[IBIS Ver]   3.2
[File Name]   sprm125.ibs
[File Rev]   0.1
[Date]   September 5, 2003
[Source]   IBIS Model Generated from PACED 4.51F
[Disclaimer]   Please be aware that in the absence of a written agreement
|   Texas Instruments(TI) assumes no liability for:
|   (1) The accuracy of the IBIS models provided to your company
|   (2) The proper functioning of these Models in your design
|   or for any resulting applications
|   (3) Infringement of patents, copyrights or intellectual
|   property rights resulting from your use of these
|   models.
|   TI provides IBIS Models as a service to our customers and
|   therefore reserves the right to limit distribution of the
|   Models.
[Copyright]   Property of Texas Instruments Incorporated.
|   Unauthorized reproduction and/or distribution is strictly.
|   prohibited.
|   This product is protected under copyright law and trade
|   secret law as an unpublished work.
|   Created 2003,(C) Copyright 1999-2003,
|   Texas Instruments Incorporated., All Rights Reserved.
|   These commodities are under the U.S. Government
|   distribution license control. As such,they are not to be
|   re-exported without the prior approval of the U.S.
|   Department of Commerce.
[Notes]
|****** ****   ***** *****   ******  Package Models  **************************
[Component]   DM641_GDK
[Manufacturer]  Texas Instruments
[Package]
|Variable  Typ   Min   Max
 R_pkg   0.12581866  0.0708   0.1927
 L_pkg   2.32E-09   1.26E-09  3.57E-09
 C_pkg   1.14E-12   6.40E-13  1.77E-12
[Pin]   signal_name  model_name   R_pin   L_pin   C_pin
B4   NMI   IT33THYPD   0.1574   2.92E-09  1.37E-12
A4   TINP0   IT33THYPD   0.1714   3.17E-09  1.50E-12
C5   TOUT0   BT3325CTPD   0.1355   2.49E-09  1.22E-12
B5   TOUT1   BT3325CTPU   0.1504   2.77E-09  1.35E-12
A5   TINP1   IT33THYPD   0.1652   3.05E-09  1.47E-12
D6   CLKOUT4   BT3315DTHYPU   0.1173   2.16E-09  1.06E-12
C6   CLKOUT6   BT3315DTHYPU   0.1352   2.50E-09  1.19E-12
A15   EMU0   BT3315DTHYPU   0.1531   2.82E-09  1.33E-12
A16   TCK   IT33THYPU   0.1598   2.93E-09  1.43E-12
C14   EMU1   BT3315DTHYPU   0.1107   2.01E-09  1.02E-12
B15   EMU2   BT3315DTHYPU   0.1318   2.37E-09  1.17E-12
C15   EMU3   BT3315DTHYPU   0.1149   2.09E-09  1.06E-12
D14   TRSTZ   IT33THYPD   0.0895   1.61E-09  8.52E-13
B16   EMU5   BT3315DTHYPU   0.1348   2.46E-09  1.21E-12
A17   EMU7   BT3315DTHYPU   0.1482   2.72E-09  1.32E-12
C16   EMU6   BT3315DTHYPU   0.1043   1.89E-09  9.63E-13
D15   EMU4   BT3315DTHYPU   0.0836   1.51E-09  7.86E-13
E15   TMS   IT33THYPU   0.0754   1.35E-09  7.23E-13
B17   EMU9   BT3315DTHYPU   0.1316   2.41E-09  1.18E-12
A18   TDI   IT33THYPU   0.1516   2.78E-09  1.35E-12
C17   EMU10   BT3315DTHYPU   0.1174   2.15E-09  1.05E-12
D16   EMU8   BT3315DTHYPU   0.093   1.70E-09  8.42E-13
B18   TDO   BT3325CTPU   0.1357   2.49E-09  1.22E-12
A20   AED13   BT3315DTPU   0.1718   3.17E-09  1.51E-12
B20   AED11   BT3315DTPU   0.1583   2.93E-09  1.39E-12
D17   EMU11   BT3315DTHYPU   0.0955   1.75E-09  8.81E-13
C19   AED15   BT3315DTPU   0.1283   2.36E-09  1.16E-12
A21   AED09   BT3315DTPU   0.174   3.21E-09  1.54E-12
C20   AED10   BT3315DTPU   0.1378   2.53E-09  1.26E-12
B21   AED07   BT3315DTPU   0.1588   2.93E-09  1.42E-12
D19   AED14   BT3315DTPU   0.1105   2.01E-09  1.04E-12
C21   AED06   BT3315DTPU   0.1445   2.64E-09  1.33E-12
B22   AED03   BT3315DTPU   0.1665   3.06E-09  1.51E-12
D20   AED12   BT3315DTPU   0.1178   2.14E-09  1.11E-12
A23   AED05   BT3315DTPU   0.1861   3.43E-09  1.67E-12
C22   AED04   BT3315DTPU   0.1485   2.71E-09  1.37E-12
D21   AED08   BT3315DTPU   0.1256   2.29E-09  1.17E-12
B23   AED02   BT3315DTPU   0.1627   3.00E-09  1.44E-12
A24   AED01   BT3315DTPU   0.1927   3.57E-09  1.68E-12
B24   AED00   BT3315DTPU   0.1784   3.29E-09  1.59E-12
C25   AED30   BT3315DTPU   0.1772   3.27E-09  1.57E-12
C26   AED31   BT3315DTPU   0.1873   3.44E-09  1.66E-12
D25   AED28   BT3315DTPU   0.161   2.97E-09  1.47E-12
D26   AED29   BT3315DTPU   0.1818   3.39E-09  1.71E-12
E25   AED26   BT3315DTPU   0.1682   3.14E-09  1.57E-12
E24   AED27   BT3315DTPU   0.1418   2.60E-09  1.29E-12
F26   AED22   BT3315DTPU   0.1743   3.21E-09  1.55E-12
F25   AED24   BT3315DTPU   0.1589   2.91E-09  1.42E-12
F24   AED25   BT3315DTPU   0.1434   2.63E-09  1.29E-12
F23   AED23   BT3315DTPU   0.1237   2.25E-09  1.12E-12
G26   AED18   BT3315DTPU   0.1471   2.70E-09  1.31E-12
G25   AED20   BT3315DTPU   0.1445   2.64E-09  1.30E-12
G24   AED21   BT3315DTPU   0.1401   2.57E-09  1.26E-12
G23   AED19   BT3315DTPU   0.1202   2.20E-09  1.08E-12
H25   AECLKIN   IT33THYPD   0.1487   2.75E-09  1.29E-12
H24   AED16   BT3315DTPU   0.1248   2.30E-09  1.09E-12
H23   AED17   BT3315DTPU   0.1074   1.97E-09  9.56E-13
J25   ASDCASZ   BT3315DTPU   0.1364   2.48E-09  1.17E-12
J24   ASDRASZ   BT3315DTPU   0.1224   2.24E-09  1.03E-12
J23   AECLKOT2   BT3315DTPD   0.1   1.86E-09  8.55E-13
J26   AECLKOT1   BT3315DTPD   0.1448   2.65E-09  1.23E-12
K23   ACE2Z   BT3315DTPU   0.0938   1.72E-09  8.52E-13
K24   ACE1Z   BT3315DTPU   0.1113   2.04E-09  1.02E-12
K25   ACE0Z   BT3315DTPU   0.1259   2.31E-09  1.15E-12
K26   ASDWEZ   BT3315DTPU   0.1406   2.59E-09  1.26E-12
L23   ABE01Z   BT3315DTPU   0.0961   1.75E-09  8.81E-13
L22   AARDY   IT33THYPU   0.0784   1.42E-09  7.32E-13
L24   ABE00Z   BT3315DTPU   0.1071   1.97E-09  9.65E-13
L25   ASDCKE   BT3315DTPU   0.125   2.30E-09  1.12E-12
L26   ACE3Z   BT3315DTPU   0.139   2.56E-09  1.23E-12
M22   APDTZ   BT3315DTPU   0.074   1.34E-09  6.98E-13
M23   AEA04   BT3315DTPD   0.0903   1.64E-09  8.30E-13
M24   AEA03   BT3315DTPD   0.105   1.91E-09  9.64E-13
M25   ABE03Z   BT3315DTPU   0.1201   2.20E-09  1.08E-12
N22   AHOLDAZ   BT3315DTPU   0.0724   1.30E-09  6.85E-13
N23   AEA07   BT3315DTPD   0.1669   3.04E-09  1.52E-12
N24   AEA06   BT3315DTPD   0.1016   1.84E-09  9.39E-13
M26   ABE02Z   BT3315DTPU   0.1409   2.59E-09  1.26E-12
N26   AEA05   BT3315DTPD   0.1326   2.42E-09  1.20E-12
P26   AEA08   BT3315DTPD   0.1329   2.42E-09  1.20E-12
P24   AEA09   BT3315DTPD   0.103   1.87E-09  9.43E-13
P23   AEA10   BT3315DTPD   0.0883   1.60E-09  8.14E-13
P22   ABUSREQ0   BT3315DTPU   0.0734   1.33E-09  6.83E-13
R24   AEA11   BT3315DTPD   0.1062   1.94E-09  9.60E-13
R23   AEA12   BT3315DTPD   0.0913   1.67E-09  8.28E-13
R22   ASOE3Z   BT3315DTPU   0.0749   1.36E-09  6.97E-13
T25   AEA13   BT3315DTPD   0.1263   2.32E-09  1.11E-12
T24   AEA14   BT3315DTPD   0.1116   2.05E-09  9.87E-13
U26   AEA15   BT3315DTPD   0.1406   2.61E-09  1.22E-12
U25   AEA16   BT3315DTPD   0.1258   2.32E-09  1.13E-12
U24   AEA17   BT3315DTPD   0.1112   2.05E-09  9.99E-13
U23   AEA22   BT3315DTPD   0.0967   1.77E-09  8.72E-13
V26   AEA19   BT3315DTPD   0.14   2.63E-09  1.28E-12
V25   AEA20   BT3315DTPD   0.1264   2.36E-09  1.16E-12
V24   AEA21   BT3315DTPD   0.1128   2.10E-09  1.03E-12
V23   AEA18   BT3315DTPD   0.0992   1.83E-09  8.94E-13
W24   AHOLDZ   IT33THYPU   0.121   2.23E-09  1.07E-12
AC17   VP0CTL1   BT3325CTHYPD   0.099   1.83E-09  9.31E-13
AD17   VP0CTL2   BT3325CTHYPD   0.1128   2.08E-09  1.03E-12
AE17   VP0CTL0   BT3325CTHYPD   0.1271   2.35E-09  1.16E-12
AF17   VP0D00   BT3325CTHYPD   0.1412   2.61E-09  1.23E-12
AB16   VP0D05   BT3325CTHYPD   0.0792   1.45E-09  7.33E-13
AC16   VP0D04   BT3325CTHYPD   0.1264   2.33E-09  1.12E-12
AD16   VP0D03   BT3325CTHYPD   0.1533   2.85E-09  1.31E-12
AE16   VP0D02   BT3325CTHYPD   0.1271   2.35E-09  1.14E-12
AD15   VP0D07   BT3325CTHYPD   0.1131   2.08E-09  1.02E-12
AF16   VP0D01   BT3325CTHYPD   0.1438   2.65E-09  1.27E-12
AE15   VP0D06   BT3325CTHYPD   0.13   2.38E-09  1.17E-12
AF14   VP0CLK0   IT33THYPD   0.1386   2.55E-09  1.24E-12
AF12   VP0CLK1   BT3325CTHYPD   0.1447   2.67E-09  1.29E-12
AB14   AHCLKR0   BT3325CTHYPD   0.0714   1.29E-09  6.76E-13
AC14   AFSR0   BT3325CTHYPD   0.092   1.68E-09  8.40E-13
AD14   ACLKR0   BT3325CTHYPD   0.1084   1.98E-09  9.80E-13
AB13   ACLKX0   BT3325CTHYPD   0.0783   1.44E-09  7.05E-13
AC13   AMUTE0   BT3325CTHYPD   0.0933   1.72E-09  8.66E-13
AD13   AMUTEIN0   BT3325CTHYPD   0.107   1.98E-09  1.01E-12
AD12   AFSX0   BT3325CTHYPD   0.1063   1.97E-09  1.00E-12
AC12   AHCLKX0   BT3325CTHYPD   0.0976   1.79E-09  8.77E-13
AE11   AXR03   BT3325CTHYPD   0.1252   2.30E-09  1.12E-12
AC10   AXR02   BT3325CTHYPD   0.1109   2.04E-09  1.01E-12
AD10   AXR01   BT3325CTHYPD   0.1261   2.32E-09  1.14E-12
AC9   AXR00   BT3325CTHYPD   0.1032   1.90E-09  9.58E-13
AF10   VP1CLK1   BT3325CTHYPD   0.1484   2.74E-09  1.32E-12
AC8   VP1D07   BT3325CTHYPD   0.0916   1.69E-09  8.54E-13
AF8   VP1CLK0   IT33THYPD   0.154   2.84E-09  1.37E-12
AD8   VP1D06   BT3325CTHYPD   0.1547   2.76E-09  1.30E-12
AE7   VP1D03   BT3325CTHYPD   0.1577   2.93E-09  1.41E-12
AC7   VP1D05   BT3325CTHYPD   0.1305   2.33E-09  1.09E-12
AD7   VP1D04   BT3325CTHYPD   0.122   2.26E-09  1.12E-12
AE6   VP1D00   BT3325CTHYPD   0.15   2.78E-09  1.38E-12
AD6   VP1D01   BT3325CTHYPD   0.1356   2.51E-09  1.25E-12
AC6   VP1D02   BT3325CTHYPD   0.1177   2.17E-09  1.10E-12
AF4   VP1CTL0   BT3325CTHYPD   0.1766   3.28E-09  1.58E-12
AE5   VP1CTL1   BT3325CTHYPD   0.1513   2.80E-09  1.39E-12
AE4   CLKMODE1   IT33THYPD   0.1584   2.95E-09  1.42E-12
AD5   VP1CTL2   BT3325CTHYPD   0.1872   3.52E-09  1.62E-12
AC2   CLKIN   IDPECLT   0.1646   3.07E-09  1.46E-12
Y4   HD2   BPCI66T   0.1033   1.92E-09  9.33E-13
AD1   VDAC   BT3325CTHYPD   0.1864   3.52E-09  1.77E-12
AC1   STCLK   IT33THYPD   0.1773   3.33E-09  1.66E-12
W4   HD6   BPCI66T   0.1035   1.90E-09  9.87E-13
Y3   HD0   BPCI66T   0.1276   2.35E-09  1.21E-12
AA2   CLKMODE0   IT33THYPD   0.151   2.80E-09  1.42E-12
W3   HD4   BPCI66T   0.1184   2.17E-09  1.16E-12
Y2   HD3   BPCI66T   0.1431   2.65E-09  1.36E-12
AA1   HD1   BPCI66T   0.1663   3.09E-09  1.52E-12
U4   HD11   BPCI66T   0.0913   1.68E-09  8.69E-13
V3   HD9   BPCI66T   0.1155   2.16E-09  1.07E-12
W2   HD7   BPCI66T   0.1409   2.63E-09  1.29E-12
U3   HD13   BPCI66T   0.1115   2.07E-09  1.05E-12
V2   HD8   BPCI66T   0.1381   2.54E-09  1.29E-12
Y1   HD5   BPCI66T   0.1775   3.29E-09  1.61E-12
T3   HD15   BPCI66T   0.1057   1.93E-09  1.00E-12
R5   MDCLK   BT3325CTHYPD   0.0731   1.31E-09  7.11E-13
U2   HD12   BPCI66T   0.1339   2.45E-09  1.24E-12
V1   HD10   BPCI66T   0.1579   2.92E-09  1.45E-12
R3   HCNTL0   BPCI66T   0.1021   1.86E-09  9.68E-13
P5   MDIO   BT3325CTPU   0.0709   1.26E-09  6.93E-13
P4   RESETZ   IT33THY   0.0874   1.58E-09  8.34E-13
T2   HDS2Z   BPCI66T   0.1346   2.47E-09  1.24E-12
U1   HD14   BPCI66T   0.1603   2.96E-09  1.46E-12
P3   HASZ   BPCI66T   0.1032   1.87E-09  9.86E-13
R2   HDS1Z   BPCI66T   0.1292   2.36E-09  1.21E-12
R1   HCSZ   BPCI66T   0.1457   2.67E-09  1.34E-12
P1   HCNTL1   BPCI66T   0.1348   2.46E-09  1.26E-12
N1   HRDYZ   BPCI66T   0.136   2.48E-09  1.27E-12
N3   HHWIL   BPCI66T   0.1   1.82E-09  9.48E-13
N4   HINTZ   BPCI66T   0.0733   1.32E-09  7.29E-13
M1   HR_WZ   BPCI66T   0.1347   2.49E-09  1.24E-12
M2   MTDX1   BPCI66T   0.1201   2.20E-09  1.14E-12
M3   MTDX0   BPCI66T   0.1055   1.94E-09  9.90E-13
M4   MTDX2   BPCI66T   0.0894   1.65E-09  8.28E-13
M5   GP0   BT3325CTHYPD   0.0753   1.38E-09  7.15E-13
L2   MTDX3   BPCI66T   0.1209   2.25E-09  1.11E-12
L3   MTXEN   BPCI66T   0.1068   1.98E-09  9.96E-13
L4   MTCLK   BPCI66T   0.0923   1.70E-09  8.70E-13
L5   GP3   BT3325CTHYPD   0.0739   1.35E-09  7.04E-13
K2   MCOL   BPCI66T   0.1253   2.32E-09  1.15E-12
K4   MRXD0   BPCI66T   0.0951   1.74E-09  9.22E-13
J1   MRXD1   BPCI66T   0.141   2.61E-09  1.32E-12
J3   MRXD2   BPCI66T   0.1124   2.06E-09  1.08E-12
J4   MRXDV   BPCI66T   0.0963   1.76E-09  9.43E-13
H2   MRXD3   BPCI66T   0.1305   2.43E-09  1.25E-12
G1   MRCLK   BPCI66T   0.1516   2.83E-09  1.41E-12
H3   MCR   BPCI66T   0.1173   2.17E-09  1.12E-12
G2   MRXER   BPCI66T   0.1373   2.55E-09  1.28E-12
F2   EXT_INT6   BT3325CTHYPU   0.1385   2.59E-09  1.24E-12
F3   EXT_INT5   BT3325CTHYPU   0.1254   2.32E-09  1.15E-12
E1   EXT_INT7   BT3325CTHYPU   0.1561   2.90E-09  1.41E-12
F4   EXT_INT4   BT3325CTHYPU   0.1061   1.97E-09  1.02E-12
D3   SDA0   BQ0001THY   0.1356   2.53E-09  1.28E-12
E4   SCL0   BQ0001THY   0.0985   1.86E-09  9.77E-13
| Reserved Pins
|V6   Reserved
|AA3   Reserved
|AD3   Reserved
|AC4   Reserved
|E14   Reserved
|AF3   Reserved
|AB3   Reserved
|C1   Reserved
|C7   Reserved
|D7   Reserved
|A7   Reserved
|D8   Reserved
|C8   Reserved
|B8   Reserved
|D9   Reserved
|C9   Reserved
|B9   Reserved
|A9   Reserved
|D10   Reserved
|C10   Reserved
|B10   Reserved
|A10   Reserved
|D11   Reserved
|E11   Reserved
|C11   Reserved
|B11   Reserved
|A11   Reserved
|E12   Reserved
|D12   Reserved
|C12   Reserved
|B12   Reserved
|E13   Reserved
|A13   Reserved
|Y26   Reserved
|Y25   Reserved
|W23   Reserved
|Y24   Reserved
|Y23   Reserved
|AA26   Reserved
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[Component]   DM641_GNZ
[Manufacturer]  Texas Instruments
[Package]
|Variable  Typ   Min   Max
 R_pkg   0.111578511  0.001847  0.2627
 L_pkg   2.35E-09   4.05E-11  5.38E-09
 C_pkg   2.25E-12   2.44E-14  4.91E-12
[Pin]   signal_name  model_name   R_pin   L_pin   C_pin
B4   NMI   IT33THYPD   0.1673   3.47E-09  3.20E-12
A4   TINP0   IT33THYPD   0.1825   3.81E-09  3.44E-12
C5   TOUT0   BT3325CTPD   0.1683   3.44E-09  3.18E-12
B5   TOUT1   BT3325CTPU   0.1829   3.73E-09  3.52E-12
A5   TINP1   IT33THYPD   0.1986   4.09E-09  3.78E-12
D6   CLKOUT4   BT3315DTHYPU   0.1719   3.53E-09  3.21E-12
C6   CLKOUT6   BT3315DTHYPU   0.1869   3.83E-09  3.54E-12
A15   EMU0   BT3315DTHYPU   0.2261   4.52E-09  4.44E-12
A16   TCK   IT33THYPU   0.2364   4.73E-09  4.68E-12
C14   EMU1   BT3315DTHYPU   0.1976   3.98E-09  3.78E-12
B15   EMU2   BT3315DTHYPU   0.2239   4.57E-09  4.35E-12
C15   EMU3   BT3315DTHYPU   0.2123   4.36E-09  4.05E-12
D14   TRSTZ   IT33THYPD   0.1813   3.67E-09  3.43E-12
B16   EMU5   BT3315DTHYPU   0.2164   4.46E-09  4.15E-12
A17   EMU7   BT3315DTHYPU   0.2223   4.54E-09  4.39E-12
C16   EMU6   BT3315DTHYPU   0.191   3.95E-09  3.89E-12
D15   EMU4   BT3315DTHYPU   0.1768   3.62E-09  3.39E-12
E15   TMS   IT33THYPU   0.1623   3.32E-09  3.02E-12
B17   EMU9   BT3315DTHYPU   0.1985   4.10E-09  3.92E-12
A18   TDI   IT33THYPU   0.2137   4.40E-09  4.17E-12
C17   EMU10   BT3315DTHYPU   0.1791   3.69E-09  3.43E-12
D16   EMU8   BT3315DTHYPU   0.1554   3.19E-09  2.92E-12
B18   TDO   BT3325CTPU   0.1886   3.93E-09  3.56E-12
A20   AED13   BT3315DTPU   0.213   4.35E-09  4.21E-12
B20   AED11   BT3315DTPU   0.1915   4.00E-09  3.66E-12
D17   EMU11   BT3315DTHYPU   0.1479   3.04E-09  2.81E-12
C19   AED15   BT3315DTPU   0.1748   3.64E-09  3.33E-12
A21   AED09   BT3315DTPU   0.2084   4.32E-09  4.13E-12
C20   AED10   BT3315DTPU   0.1779   3.70E-09  3.48E-12
B21   AED07   BT3315DTPU   0.1939   4.06E-09  3.71E-12
D19   AED14   BT3315DTPU   0.1442   2.99E-09  2.76E-12
C21   AED06   BT3315DTPU   0.1698   3.57E-09  3.27E-12
B22   AED03   BT3315DTPU   0.197   4.19E-09  3.76E-12
D20   AED12   BT3315DTPU   0.1424   2.99E-09  2.74E-12
A23   AED05   BT3315DTPU   0.2017   4.18E-09  4.14E-12
C22   AED04   BT3315DTPU   0.1637   3.43E-09  3.30E-12
D21   AED08   BT3315DTPU   0.1414   2.95E-09  2.85E-12
B23   AED02   BT3315DTPU   0.1795   3.78E-09  3.62E-12
A24   AED01   BT3315DTPU   0.1949   4.13E-09  3.94E-12
B24   AED00   BT3315DTPU   0.1806   3.85E-09  3.65E-12
C25   AED30   BT3315DTPU   0.1751   3.73E-09  3.56E-12
C26   AED31   BT3315DTPU   0.1812   3.84E-09  3.71E-12
D25   AED28   BT3315DTPU   0.1588   3.41E-09  3.19E-12
D26   AED29   BT3315DTPU   0.1535   3.32E-09  2.98E-12
E25   AED26   BT3315DTPU   0.1392   3.01E-09  2.85E-12
E24   AED27   BT3315DTPU   0.1235   2.66E-09  2.59E-12
F26   AED22   BT3315DTPU   0.1359   2.90E-09  2.87E-12
F25   AED24   BT3315DTPU   0.1218   2.60E-09  2.57E-12
F24   AED25   BT3315DTPU   0.1081   2.33E-09  2.24E-12
F23   AED23   BT3315DTPU   0.09372   2.03E-09  1.90E-12
G26   AED18   BT3315DTPU   0.1307   2.79E-09  2.74E-12
G25   AED20   BT3315DTPU   0.117   2.51E-09  2.43E-12
G24   AED21   BT3315DTPU   0.1038   2.24E-09  2.10E-12
G23   AED19   BT3315DTPU   0.08718   1.87E-09  1.77E-12
H25   AECLKIN   IT33THYPD   0.1085   2.26E-09  2.32E-12
H24   AED16   BT3315DTPU   0.09543   2.00E-09  2.00E-12
H23   AED17   BT3315DTPU   0.07998   1.72E-09  1.65E-12
J25   ASDCASZ   BT3315DTPU   0.1025   2.19E-09  2.18E-12
J24   ASDRASZ   BT3315DTPU   0.08962   1.87E-09  1.94E-12
J23   AECLKOT2   BT3315DTPD   0.06798   1.40E-09  1.53E-12
J26   AECLKOT1   BT3315DTPD   0.09615   1.98E-09  2.17E-12
K23   ACE2Z   BT3315DTPU   0.04876   1.01E-09  1.07E-12
K24   ACE1Z   BT3315DTPU   0.0604   1.28E-09  1.32E-12
K25   ACE0Z   BT3315DTPU   0.07216   1.52E-09  1.59E-12
K26   ASDWEZ   BT3315DTPU   0.08386   1.76E-09  1.85E-12
L23   ABE01Z   BT3315DTPU   0.04507   9.45E-10  9.91E-13
L22   AARDY   IT33THYPU   0.02986   6.45E-10  6.36E-13
L24   ABE00Z   BT3315DTPU   0.05386   1.14E-09  1.17E-12
L25   ASDCKE   BT3315DTPU   0.06558   1.39E-09  1.41E-12
L26   ACE3Z   BT3315DTPU   0.07756   1.65E-09  1.63E-12
M22   APDTZ   BT3315DTPU   0.01512   3.11E-10  3.27E-13
M23   AEA04   BT3315DTPD   0.02738   5.70E-10  5.90E-13
M24   AEA03   BT3315DTPD   0.01819   3.70E-10  3.93E-13
M25   ABE03Z   BT3315DTPU   0.01965   3.98E-10  4.08E-13
N22   AHOLDAZ   BT3315DTPU   0.02843   6.39E-10  5.35E-13
N23   AEA07   BT3315DTPD   0.04193   9.12E-10  8.78E-13
N24   AEA06   BT3315DTPD   0.05535   1.19E-09  1.19E-12
M26   ABE02Z   BT3315DTPU   0.09055   1.89E-09  1.99E-12
N26   AEA05   BT3315DTPD   0.08206   1.74E-09  1.81E-12
P26   AEA08   BT3315DTPD   0.08239   1.74E-09  1.80E-12
P24   AEA09   BT3315DTPD   0.05887   1.25E-09  1.28E-12
P23   AEA10   BT3315DTPD   0.04708   1.04E-09  9.24E-13
P22   ABUSREQ0   BT3315DTPU   0.03785   8.32E-10  7.51E-13
R24   AEA11   BT3315DTPD   0.06489   1.36E-09  1.41E-12
R23   AEA12   BT3315DTPD   0.05301   1.12E-09  1.13E-12
R22   ASOE3Z   BT3315DTPU   0.0412   8.50E-10  8.74E-13
T25   AEA13   BT3315DTPD   0.08306   1.70E-09  1.78E-12
T24   AEA14   BT3315DTPD   0.07127   1.53E-09  1.50E-12
U26   AEA15   BT3315DTPD   0.1015   2.20E-09  2.03E-12
U25   AEA16   BT3315DTPD   0.08964   1.93E-09  1.87E-12
U24   AEA17   BT3315DTPD   0.07784   1.69E-09  1.60E-12
U23   AEA22   BT3315DTPD   0.06592   1.42E-09  1.36E-12
V26   AEA19   BT3315DTPD   0.1074   2.31E-09  2.19E-12
V25   AEA20   BT3315DTPD   0.09563   2.03E-09  2.03E-12
V24   AEA21   BT3315DTPD   0.08386   1.78E-09  1.78E-12
V23   AEA18   BT3315DTPD   0.07183   1.53E-09  1.53E-12
W24   AHOLDZ   IT33THYPU   0.103   2.20E-09  2.17E-12
AC17   VP0CTL1   BT3325CTHYPD   0.06316   1.36E-09  1.29E-12
AD17   VP0CTL2   BT3325CTHYPD   0.07514   1.62E-09  1.55E-12
AE17   VP0CTL0   BT3325CTHYPD   0.08605   1.86E-09  1.78E-12
AF17   VP0D00   BT3325CTHYPD   0.09961   2.16E-09  1.96E-12
AB16   VP0D05   BT3325CTHYPD   0.04359   9.41E-10  8.56E-13
AC16   VP0D04   BT3325CTHYPD   0.04748   1.03E-09  9.25E-13
AD16   VP0D03   BT3325CTHYPD   0.05847   1.27E-09  1.19E-12
AE16   VP0D02   BT3325CTHYPD   0.0752   1.64E-09  1.51E-12
AD15   VP0D07   BT3325CTHYPD   0.06037   1.32E-09  1.23E-12
AF16   VP0D01   BT3325CTHYPD   0.1001   2.15E-09  2.05E-12
AE15   VP0D06   BT3325CTHYPD   0.0811   1.75E-09  1.67E-12
AF14   VP0CLK0   IT33THYPD   0.08342   1.71E-09  1.79E-12
AF12   VP0CLK1   BT3325CTHYPD   0.06122   1.27E-09  1.36E-12
AB14   AHCLKR0   BT3325CTHYPD   0.05532   1.20E-09  1.15E-12
AC14   AFSR0   BT3325CTHYPD   0.05336   1.18E-09  1.05E-12
AD14   ACLKR0   BT3325CTHYPD   0.0611   1.30E-09  1.28E-12
AB13   ACLKX0   BT3325CTHYPD   0.05761   1.21E-09  1.28E-12
AC13   AMUTE0   BT3325CTHYPD   0.05522   1.18E-09  1.21E-12
AD13   AMUTEIN0   BT3325CTHYPD   0.06896   1.47E-09  1.51E-12
AD12   AFSX0   BT3325CTHYPD   0.06935   1.48E-09  1.52E-12
AC12   AHCLKX0   BT3325CTHYPD   0.0618   1.36E-09  1.27E-12
AE11   AXR03   BT3325CTHYPD   0.0772   1.64E-09  1.68E-12
AC10   AXR02   BT3325CTHYPD   0.07778   1.65E-09  1.81E-12
AD10   AXR01   BT3325CTHYPD   0.09011   1.94E-09  1.99E-12
AC9   AXR00   BT3325CTHYPD   0.06988   1.52E-09  1.48E-12
AF10   VP1CLK1   BT3325CTHYPD   0.09702   1.93E-09  2.10E-12
AC8   VP1D07   BT3325CTHYPD   0.07397   1.58E-09  1.60E-12
AF8   VP1CLK0   IT33THYPD   0.1186   2.45E-09  2.62E-12
AD8   VP1D06   BT3325CTHYPD   0.1188   2.48E-09  2.53E-12
AE7   VP1D03   BT3325CTHYPD   0.1092   2.31E-09  2.32E-12
AC7   VP1D05   BT3325CTHYPD   0.08554   1.85E-09  1.85E-12
AD7   VP1D04   BT3325CTHYPD   0.1025   2.22E-09  2.18E-12
AE6   VP1D00   BT3325CTHYPD   0.1175   2.57E-09  2.48E-12
AD6   VP1D01   BT3325CTHYPD   0.1059   2.31E-09  2.24E-12
AC6   VP1D02   BT3325CTHYPD   0.09416   2.05E-09  2.01E-12
AF4   VP1CTL0   BT3325CTHYPD   0.1458   3.16E-09  3.04E-12
AE5   VP1CTL1   BT3325CTHYPD   0.136   2.95E-09  2.91E-12
AE4   CLKMODE1   IT33THYPD   0.1296   2.86E-09  2.64E-12
AD5   VP1CTL2   BT3325CTHYPD   0.1457   3.12E-09  2.96E-12
AC2   CLKIN   IDPECLT   0.1335   2.67E-09  2.29E-12
Y4   HD2   BPCI66T   0.06144   1.27E-09  1.32E-12
AD1   VDAC   BT3325CTHYPD   0.1272   2.74E-09  2.66E-12
AC1   STCLK   IT33THYPD   0.1178   2.60E-09  2.37E-12
W4   HD6   BPCI66T   0.05967   1.30E-09  1.29E-12
Y3   HD0   BPCI66T   0.07939   1.75E-09  1.66E-12
AA2   CLKMODE0   IT33THYPD   0.09906   2.17E-09  2.04E-12
W3   HD4   BPCI66T   0.0695   1.52E-09  1.50E-12
Y2   HD3   BPCI66T   0.08944   2.03E-09  1.70E-12
AA1   HD1   BPCI66T   0.1046   2.25E-09  2.16E-12
U4   HD11   BPCI66T   0.0409   9.03E-10  8.61E-13
V3   HD9   BPCI66T   0.06062   1.35E-09  1.23E-12
W2   HD7   BPCI66T   0.07874   1.73E-09  1.53E-12
U3   HD13   BPCI66T   0.05242   1.17E-09  1.02E-12
V2   HD8   BPCI66T   0.07134   1.56E-09  1.44E-12
Y1   HD5   BPCI66T   0.1037   2.19E-09  2.14E-12
T3   HD15   BPCI66T   0.04306   9.77E-10  8.02E-13
R5   MDCLK   BT3325CTHYPD   0.01076   2.41E-10  2.07E-13
U2   HD12   BPCI66T   0.06139   1.35E-09  1.23E-12
V1   HD10   BPCI66T   0.08047   1.71E-09  1.66E-12
R3   HCNTL0   BPCI66T   0.03397   7.71E-10  6.25E-13
P5   MDIO   BT3325CTPU   0.001847  4.05E-11  2.44E-14
P4   RESETZ   IT33THY   0.03695   8.40E-10  7.26E-13
T2   HDS2Z   BPCI66T   0.0773   1.72E-09  1.59E-12
U1   HD14   BPCI66T   0.09881   2.09E-09  2.13E-12
P3   HASZ   BPCI66T   0.05249   1.13E-09  1.16E-12
R2   HDS1Z   BPCI66T   0.07593   1.60E-09  1.71E-12
R1   HCSZ   BPCI66T   0.08081   1.71E-09  1.80E-12
P1   HCNTL1   BPCI66T   0.08016   1.72E-09  1.77E-12
N1   HRDYZ   BPCI66T   0.07788   1.67E-09  1.75E-12
N3   HHWIL   BPCI66T   0.05455   1.23E-09  1.09E-12
N4   HINTZ   BPCI66T   0.04677   1.04E-09  9.19E-13
M1   HR_WZ   BPCI66T   0.08441   1.80E-09  1.87E-12
M2   MTDX1   BPCI66T   0.07279   1.55E-09  1.60E-12
M3   MTDX0   BPCI66T   0.06113   1.31E-09  1.34E-12
M4   MTDX2   BPCI66T   0.04961   1.09E-09  1.00E-12
M5   GP0   BT3325CTHYPD   0.0417   9.07E-10  8.11E-13
L2   MTDX3   BPCI66T   0.07932   1.70E-09  1.69E-12
L3   MTXEN   BPCI66T   0.06685   1.46E-09  1.42E-12
L4   MTCLK   BPCI66T   0.05546   1.20E-09  1.17E-12
L5   GP3   BT3325CTHYPD   0.04416   9.58E-10  8.94E-13
K2   MCOL   BPCI66T   0.05557   1.19E-09  1.12E-12
K4   MRXD0   BPCI66T   0.05188   1.12E-09  1.03E-12
J1   MRXD1   BPCI66T   0.09711   2.06E-09  1.96E-12
J3   MRXD2   BPCI66T   0.08232   1.77E-09  1.68E-12
J4   MRXDV   BPCI66T   0.07043   1.54E-09  1.38E-12
H2   MRXD3   BPCI66T   0.1007   2.18E-09  1.99E-12
G1   MRCLK   BPCI66T   0.1195   2.52E-09  2.50E-12
H3   MCR   BPCI66T   0.07266   1.59E-09  1.39E-12
G2   MRXER   BPCI66T   0.112   2.40E-09  2.20E-12
F2   EXT_INT6   BT3325CTHYPU   0.1179   2.53E-09  2.29E-12
F3   EXT_INT5   BT3325CTHYPU   0.106   2.25E-09  2.09E-12
E1   EXT_INT7   BT3325CTHYPU   0.1355   2.85E-09  2.69E-12
F4   EXT_INT4   BT3325CTHYPU   0.09476   2.01E-09  1.85E-12
D3   SDA0   BQ0001THY   0.1305   2.77E-09  2.57E-12
E4   SCL0   BQ0001THY   0.1039   2.18E-09  2.01E-12
| Models and submodels in the file (13): BPCI66T (I/O), IT33THY (Input), IT33THYPD (Input), IT33THYPU (Input), BT3315DTPU (I/O), BT3315DTPD (I/O), BT3315DTHYPU (I/O), BT3325CTPD (I/O), BT3325CTPU (I/O), BT3325CTHYPD (I/O), BT3325CTHYPU (I/O), IDPECLT (Input), BQ0001THY (I/O)
